FUNCTION_BLOCK FB92
TITLE =Get Disable State
//*****************************************************************************
//* maxon motor ag
//* R&D
//* all rights reserved
//*****************************************************************************
//* Summary:  Read device status
//*
//* Remarks:
//*
//* Created under: STEP7 REV5.2+SP1
//*****************************************************************************
//* History:
//* 19.05.2004 | INA   first release
//*
//*
//*****************************************************************************
//

AUTHOR:INA
FAMILY:StateMac
NAME:GetDisSt
VERSION:00.01


VAR_INPUT

Read : BOOL //A rising edge start the command

  NodeID : BYTE //Adress of the maxon device

END_VAR
VAR_OUTPUT
  Done : BOOL //Data valid flag is TRUE if data were available

  Err : BOOL //Error flag is TRUE if an Error has occured, see ErrNo for more details

  ErrNo : DINT //Contains detailed error information

  IsDisabled : BOOL //Device disable state

END_VAR
VAR
  xEdgeMerker : BOOL //Edge Merker

  xEdgeFlag : BOOL //Edge Flag

  xStep : INT
  xStatusword : WORD
  xNotReadyToSwitchOn : WORD
  xSwitchOnDisabled : WORD  := W#16#40
  xReadyToSwitchOn : WORD  := W#16#21
  xSwitchedOn : WORD  := W#16#23
  xFault : WORD  := W#16#8
END_VAR

BEGIN

NETWORK
TITLE = Activate the service function
//

// SDO Read "Get Disable State"

       U    #Read
       FP   #xEdgeFlag                   // recognize a positiv edge of the Read signal
       =    #xEdgeMerker                 // and set the xEdgeMerker for one cycle to true

       L    #xStep
       L    0
       ==I
       U    #xEdgeMerker
       SPB  nstp                         // iStep = 1 -> fnc1

       L    #xStep                       // jump list
       SPL  List
       SPA  rdef
       SPA  fnc1
       SPA  fncE
List  :SPA  rdef

rdef  :NOP  0
       R    #Done                        // reset Done
       R    #Err                         // reset Error
       L    0
       T    #xStep                       // iStep = 0
       SPA  end

fnc1  :NOP  0
       CALL FC1
         NodeID:=#NodeID
         Index:=DW#16#00006041
         SubIndex:=DW#16#00000000
         RET_VAL:=#Done
         Err:=#Err
         ErrNo:=#ErrNo

       L    DB219.DBW10
       UW   W#16#007F
       T    #xStatusword

       L    #xStatusword
       L    #xNotReadyToSwitchOn
       ==I
       SPB  tdis

       L    #xStatusword
       L    #xSwitchOnDisabled
       ==I
       SPB  tdis

       L    #xStatusword
       L    #xReadyToSwitchOn
       ==I
       SPB  tdis

       L    #xStatusword
       L    #xSwitchedOn
       ==I
       SPB  tdis

       L    #xStatusword
       L    #xFault
       ==I
       SPB  tdis
       SPA  fdis

tdis  :NOP  0
       S    #IsDisabled                  // set IsDisabled
       SPA  fncE

fdis  :NOP  0
       R    #IsDisabled                  // reset IsDisabled

fncE  :NOP  0
       L    0
       T    #xStep
       SPA  end

nstp  :NOP  0
       L    #xStep
       INC            1
       T    #xStep

end   :NOP  0
END_FUNCTION_BLOCK
